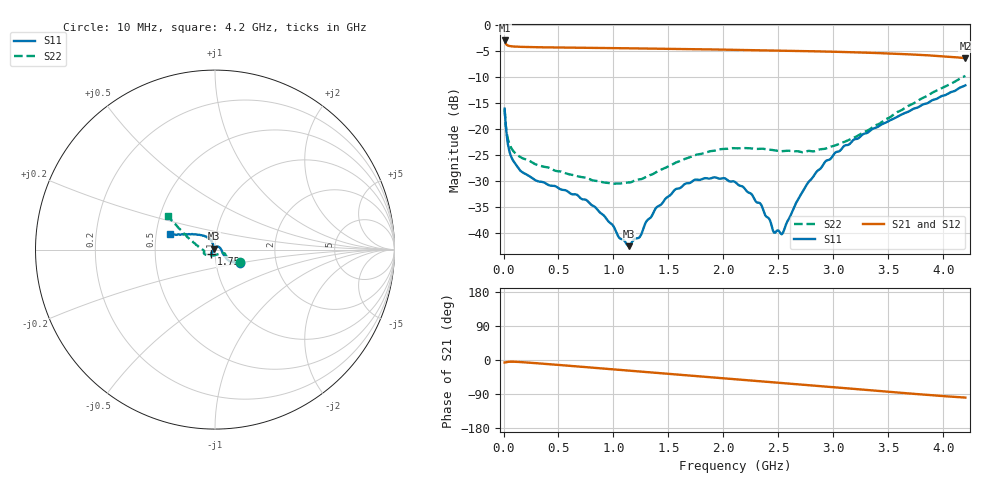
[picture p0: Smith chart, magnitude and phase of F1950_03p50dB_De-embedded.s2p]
! Integrated Device Technology
! Corporate Headquarters
! 6024 Silver Creek Valley Road
! San Jose, CA 95138  USA
! Phone:  1-408-284-8200
! Toll Free:  1-800-223-1366
! Webpage:  http://www.idt.com/
! Timing and RF Division
! 515 Groton Road, Suite 102
! Westford, MA 01886-6024
! Device:  F1950
! Description: 7-bit 0.25 dB Digital Step Attenuator
! Frequency:  150.0 -  4000.00 MHz
! Package:  4x4 mm Thin QFN Plastic Package: 24 pin
! Ports:  2 RF, 12 DC
!  Pin  1  = D0
!  Pin  2  = VDD
!  Pin  3  = Vmode
!  Pin  4  = GND
!  Pin  5  = RF1  =  Port 1
!  Pin  6  = GND
!  Pin  7  = GND
!  Pin  8  = GND
!  Pin  9  = GND
!  Pin 10  = GND
!  Pin 11  = GND
!  Pin 12  = GND
!  Pin 13  = GND
!  Pin 14  = RF2  =  Port 2
!  Pin 15  = GND
!  Pin 16  = LE
!  Pin 17  = CLK
!  Pin 18  = DATE
!  Pin 19  = D6
!  Pin 20  = D5
!  Pin 21  = D4
!  Pin 22  = D3
!  Pin 23  = D2
!  Pin 24  = D1
! State:  14
! Atten State:  3.50 dB
! Voltage:  +5.00 Volts
! Current:  Not Measured mA
! Data:  The device was measured on a the F195X evaluation board which has
!  individual transmission lines to the RF pins.  Data was collected
!  using a calibrated network analyzer.  The evaluation board was
!  de-embedded using a TRL calibration technique.
!  The reference plane is the edge of the package pin.
! Misc:  Board 2019
!  Action Tracker AT0250
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# GHz S dB R 50
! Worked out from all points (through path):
!   420 points, 10 MHz to 4.2 GHz, reference 50 ohm
!   highest |S21| = -3.04 dB at 10 MHz (marker M1); lowest = -6.4 dB at 4.2 GHz (marker M2)
!   group delay of S21, straight-line fit = 65.1 ps
!   lowest |S11| = -42.4 dB at 1.14 GHz (marker M3), VSWR 1.02, Z = 49.4 + j0.489 ohm
!   |S11| at or under -10 dB: start of sweep to end of sweep
!   |S22| runs from -30.5 to -9.8 dB; largest |S21 - S12| = 0.00075
!   S11 on the Smith chart (normalised r, x): 10 MHz: 1.30, -0.20; 1.75 GHz: 0.96, -0.05; 4.2 GHz: 0.60, +0.11
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0.01  -16.11 -28.8  -3.04 -6.6  -3.03 -6.6  -16.23 -27.6
0.06  -24.75 -32.1  -4.12 -4.5  -4.12 -4.5  -23.19 -28.4
0.15  -27.91 -15.5  -4.25 -5.3  -4.25 -5.3  -25.32 -21.5
0.71  -33.39 51.2  -4.43 -17.9  -4.43 -17.9  -29.21 -38.7
0.91  -36.51 74.0  -4.48 -22.5  -4.48 -22.6  -30.21 -56.9
1.05  -40.78 101.6  -4.52 -25.8  -4.52 -25.8  -30.44 -76.5
1.14  -42.44 139.1  -4.54 -27.9  -4.54 -27.9  -30.25 -89.3
1.24  -40.65 178.9  -4.56 -30.2  -4.56 -30.2  -29.63 -102.4
1.3  -37.67 -163.4  -4.58 -31.6  -4.58 -31.7  -29.11 -111.4
1.41  -34.75 -148.8  -4.61 -34.2  -4.61 -34.2  -28.00 -123.5
1.56  -31.61 -139.3  -4.65 -37.7  -4.65 -37.8  -26.49 -136.3
1.75  -29.67 -131.5  -4.71 -42.2  -4.71 -42.2  -24.94 -147.6
1.92  -29.25 -128.2  -4.77 -46.2  -4.76 -46.3  -24.14 -155.0
2.11  -30.22 -126.6  -4.83 -50.7  -4.83 -50.7  -23.70 -160.0
2.34  -34.39 -137.2  -4.92 -56.1  -4.92 -56.1  -23.76 -164.3
2.46  -39.85 -168.0  -4.96 -58.8  -4.96 -58.9  -24.07 -165.6
2.53  -40.17 160.7  -4.99 -60.5  -4.98 -60.5  -24.25 -167.6
2.68  -33.40 117.4  -5.04 -64.1  -5.04 -64.1  -24.27 -169.8
2.81  -29.31 110.1  -5.10 -67.2  -5.10 -67.2  -24.28 -173.7
3.1  -23.20 117.4  -5.25 -74.2  -5.25 -74.3  -22.46 177.2
3.51  -18.39 136.7  -5.53 -84.1  -5.53 -84.1  -17.80 161.1
4.2  -11.64 161.3  -6.42 -99.1  -6.42 -99.2  -9.82 144.5
